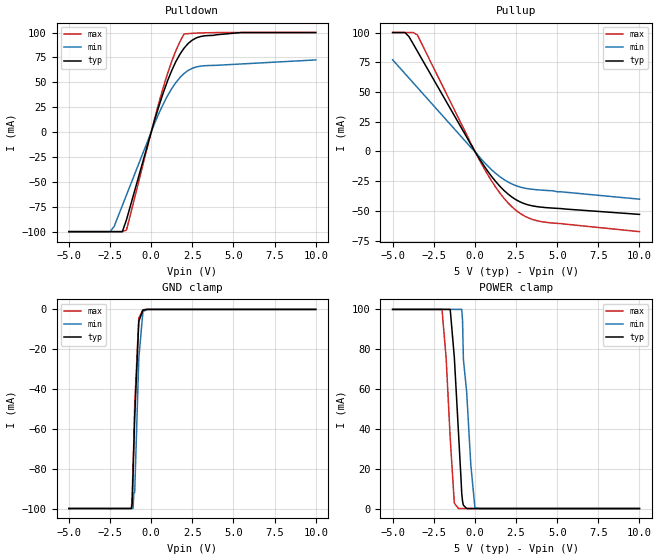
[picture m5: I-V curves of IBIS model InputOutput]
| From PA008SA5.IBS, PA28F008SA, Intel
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|**************************Input Output Model*********************************
[Model]   InputOutput
Model_type   I/O
|   for DQ[7:0]
Vinl = 0.8V
Vinh = 2.0V
| Variable   typ   min   max
C_comp   9.61p   NA   11.6p
[Voltage Range]   5.0V   4.5V   5.5V
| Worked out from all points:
|   slope of the pulldown table from 0 to 0.75 V, typ, clamps not added: 18.6 ohm
|   slope of the pullup table from 0 to 0.75 V, typ, clamps not added: 46.8 ohm
|   GND clamp passes 1 mA (typ) near -0.53 V on its own axis
|   POWER clamp passes 1 mA (typ) near -0.62 V on its own axis
[Pulldown]
| [Pullup] and [Pulldown] IV curves include only the current through
| the channels of output driver transistors when outputs are enabled
| with OE# = VIL.  Although the output driver transistors have np and
| pn diodes inherently created by CMOS IC fabrication between the
| drain and bulk of n-channel and p-channel CMOS transistors,
| the current through these junction diodes is not included in
| [Pullup] or [Pulldown].  Instead that drain/bulk diode current is
| included in the [POWER_clamp] or [GND_clamp] sections, which are
| not dependent on the state of OE# or output data value.
|Voltage  I(typ)   I(min)   I(max)
-5V       -100mA     -100mA     -100mA
-2.5V     -100mA     -100mA     -100mA
-2.25V    -100mA     -94.81mA   -100mA
-1.75V    -100mA     -73.76mA   -100mA
-1.5V     -88.1mA    -63.23mA   -98.45mA
250mV     14.17mA    10.34mA    15.97mA
750mV     40.16mA    28.7mA     45.67mA
1.5V      70.76mA    49.76mA    81.73mA
2V        84.33mA    58.89mA    98.56mA
2.5V      92.41mA    64.11mA    99.17mA
3.25V     96.69mA    66.67mA    99.7mA
10V       100mA      72.5mA     100mA
[GND_clamp]
| [POWER_clamp] and [GND_clamp] IV curves describe ESD protection
| circuits PLUS some np and pn diodes which exist between the
| drain and bulk of n-channel and p-channel CMOS transistors.
| These drain/bulk diodes are inherent in CMOS IC fabrication,
| and are visible on the node of the I/O pin at all times.
| Even the drain/bulk diodes of output driver [Pullup] and [Powerdown]
| transistors are included in [POWER_clamp] or [GND_clamp], because
| these diodes contribute to I/O pin current even when the
| chip outputs are tristated by OE# = VIH.
| For example, when V forced on the I/O pin is large, we are
| forward biasing the pn diode at the drain/bulk interface in the
| p-channel pullup transistor.  Similarly, when V forced on the
| I/O pin is sufficiently negative with respect to the substrate
| ground, we are forward biasing the np diode at the drain/bulk
| interface in the n-channel pulldown transistor.  The effects
| of these diodes are included in [POWER_clamp] or [GND_clamp].
|Voltage  I(typ)   I(min)   I(max)
-5V       -99.85mA   -99.84mA   -99.85mA
-1.2V     -99.84mA   -99.84mA   -99.85mA
-1.15V    -97.35mA   -99.84mA   -93.17mA
-1.1V     -82.77mA   -99.84mA   -77.65mA
-1.05V    -68.37mA   -91.8mA    -65.56mA
-1V       -53.99mA   -91.8mA    -48.05mA
-750mV    -5.958mA   -24.58mA   -4.306mA
-500mV    -344.6uA   -1.004mA   -201.4uA
-250mV    0A         0A         0A
10V       0A         0A         0A
[Pullup]
| (Voltages for [Pullup] and [POWER_clamp] are specified with
| negative respect to Vcc.  Reference the IBIS documentation
| for more information regarding Vtable = Vcc - Voutput.
| This method keeps -Vds constant for the values in all three
| columns across a line of the table.
| [Pullup] and [Pulldown] IV curves include only the current through
| the channels of output driver transistors when outputs are enabled
| with OE# = VIL.  Although the output driver transistors have np and
| pn diodes inherently created by CMOS IC fabrication between the
| drain and bulk of n-channel and p-channel CMOS transistors,
| the current through these junction diodes is not included in
| [Pullup] or [Pulldown].  Instead that drain/bulk diode current is
| included in the [POWER_clamp] or [GND_clamp] sections, which are
| not dependent on the state of OE# or output data value.
|Voltage  I(typ)   I(min)   I(max)
-5V       100mA      77.1mA     100mA
-4.25V    100mA      65.48mA    100mA
-4V       96.44mA    61.6mA     100mA
-3.75V    90.42mA    57.73mA    100mA
-3.5V     84.39mA    53.85mA    98.08mA
0V        0A         0A         0A
500mV     -10.94mA   -8.152mA   -12.79mA
1.5V      -29.01mA   -21.02mA   -34.64mA
2.5V      -40.6mA    -28.8mA    -49.53mA
3.25V     -44.95mA   -31.38mA   -55.86mA
4V        -46.77mA   -32.44mA   -58.88mA
10V       -52.9mA    -40.1mA    -67.4mA
[POWER_clamp]
| (Voltages for [Pullup] and [POWER_clamp] are specified with
| negative respect to Vcc.  Reference the IBIS documentation
| for more information regarding Vtable = Vcc - Voutput.
| This method keeps -Vds constant for the values in all three
| columns across a line of the table.
| [POWER_clamp] and [GND_clamp] IV curves describe ESD protection
| circuits PLUS some np and pn diodes which exist between the
| drain and bulk of n-channel and p-channel CMOS transistors.
| These drain/bulk diodes are inherent in CMOS IC fabrication,
| and are visible on the node of the I/O pin at all times.
| Even the drain/bulk diodes of output driver [Pullup] and [Powerdown]
| transistors are included in [POWER_clamp] or [GND_clamp], because
| these diodes contribute to I/O pin current even when the
| chip outputs are tristated by OE# = VIH.
| For example, when V forced on the I/O pin is large, we are
| forward biasing the pn diode at the drain/bulk interface in the
| p-channel pullup transistor.  Similarly, when V forced on the
| I/O pin is sufficiently negative with respect to the substrate
| ground, we are forward biasing the np diode at the drain/bulk
| interface in the n-channel pulldown transistor.  The effects
| of these diodes are included in [POWER_clamp] or [GND_clamp].
|Voltage  I(typ)   I(min)   I(max)
-5V       100mA      100mA      100mA
-2V       100mA      100mA      100mA
-1.75V    100mA      100mA      75.82mA
-1.5V     100mA      100mA      35.28mA
-1.25V    75.87mA    100mA      2.678mA
-1V       38.44mA    100mA      37.11nA
-800mV    7.521mA    100mA      0A
-750mV    3.623mA    94.38mA    0A
-700mV    1.661mA    75mA       0A
-250mV    0A         22.09mA    0A
0V        0A         457.4uA    0A
10V       0A         0A         0A
[Ramp]
| The DQ Ramp information is not provided at this time for the
| device but will be available in the future.  The table below
| is for the compatibility with some IBIS parsers.
| Variable   typ   min   max
 dV/dt_r   0V/0ns   0V/0ns   0V/0ns
 dV/dt_f   0V/0ns   0V/0ns   0V/0ns
